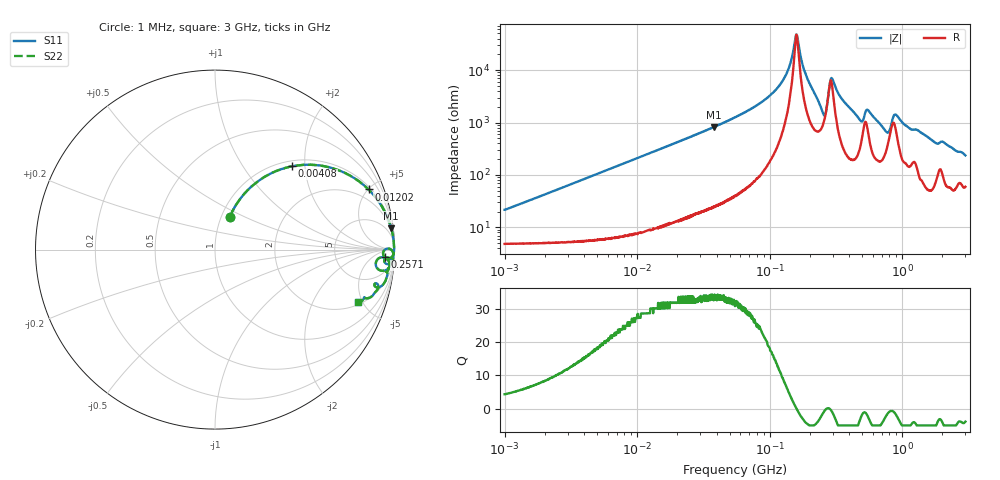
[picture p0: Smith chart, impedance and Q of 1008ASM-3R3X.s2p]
!s-Parameter Generated by FASTRON Sdn. Bhd.
!FASTRON P/N : 1008ASM-3R3X
!Keysight Technologies: E4991B_MY54100416_A.01.15
!Date: Wed Jun 19 14:52:46 2024
!Version  :Rev00  Wed Jun 19 14:52:46 2024
!Data & Calibration Information:
!Freq  S11  S21  S12  S22
!PortZ  Port1:50+j0  Port2:50+j0
!When reading reference impedance value at option line is always used.
! Remarks : This data is being provided solely for informational purposes.
# Hz S dB R 50
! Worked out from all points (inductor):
!   1601 points, 1 MHz to 3 GHz, reference 50 ohm
!   read as one part in series: L = 3.35 uH near 1.041 MHz
!   highest Q = 33.7 at 38.01 MHz (marker M1), where L = 3.44 uH
!   self-resonance near 159 MHz
!   S11 on the Smith chart (normalised r, x): 1 MHz: 1.10, +0.42; 4.08 MHz: 1.11, +1.71; 12.02 MHz: 1.17, +5.03; 257.1 MHz: 22, -18; 3 GHz: 2.19, -4.57
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1000000  -13.90 65.7  -0.58 -11.4  -0.58 -11.4  -13.90 65.7
3804036  -4.38 49.0  -2.42 -37.1  -2.42 -37.1  -4.38 49.0
4080087  -4.00 47.3  -2.65 -39.0  -2.65 -39.0  -4.00 47.3
1.202488e7  -0.74 21.4  -8.75 -66.6  -8.75 -66.6  -0.74 21.4
1.447069e7  -0.53 18.1  -10.20 -70.0  -10.20 -70.0  -0.53 18.1
3.801167e7  -0.09 6.9  -18.40 -81.4  -18.40 -81.4  -0.09 6.9
5.504702e7  -0.05 4.5  -22.10 -83.7  -22.10 -83.7  -0.05 4.5
1.171891e8  -0.02 1.2  -33.80 -84.0  -33.80 -84.0  -0.02 1.2
1.382301e8  -0.02 0.5  -40.30 -78.6  -40.30 -78.6  -0.02 0.5
1.590202e8  -0.02 0.0  -53.60 -7.3  -53.60 -7.3  -0.02 0.0
1.820241e8  -0.02 -0.5  -40.10 74.0  -40.10 74.0  -0.02 -0.5
2.083556e8  -0.04 -1.2  -33.10 77.7  -33.10 77.7  -0.04 -1.2
2.570867e8  -0.48 -2.6  -23.20 37.8  -23.20 37.8  -0.48 -2.6
2.662515e8  -0.53 -0.3  -24.60 5.6  -24.60 5.6  -0.53 -0.3
2.957531e8  -0.09 -0.6  -36.90 41.8  -36.90 41.8  -0.09 -0.6
3.48855e8  -0.05 -2.0  -29.20 80.2  -29.20 80.2  -0.05 -2.0
4.805402e8  -0.25 -4.8  -21.20 68.3  -21.20 68.3  -0.25 -4.8
5.528145e8  -0.20 -3.0  -24.90 64.7  -24.90 64.7  -0.20 -3.0
7.925923e8  -0.91 -5.6  -17.30 40.5  -17.30 40.5  -0.91 -5.6
8.937307e8  -0.33 -3.3  -23.40 55.3  -23.40 55.3  -0.33 -3.3
1.153559e9  -0.29 -7.2  -17.90 71.6  -17.90 71.6  -0.29 -7.2
3e9  -1.44 -20.3  -8.90 55.1  -8.90 55.1  -1.44 -20.3
